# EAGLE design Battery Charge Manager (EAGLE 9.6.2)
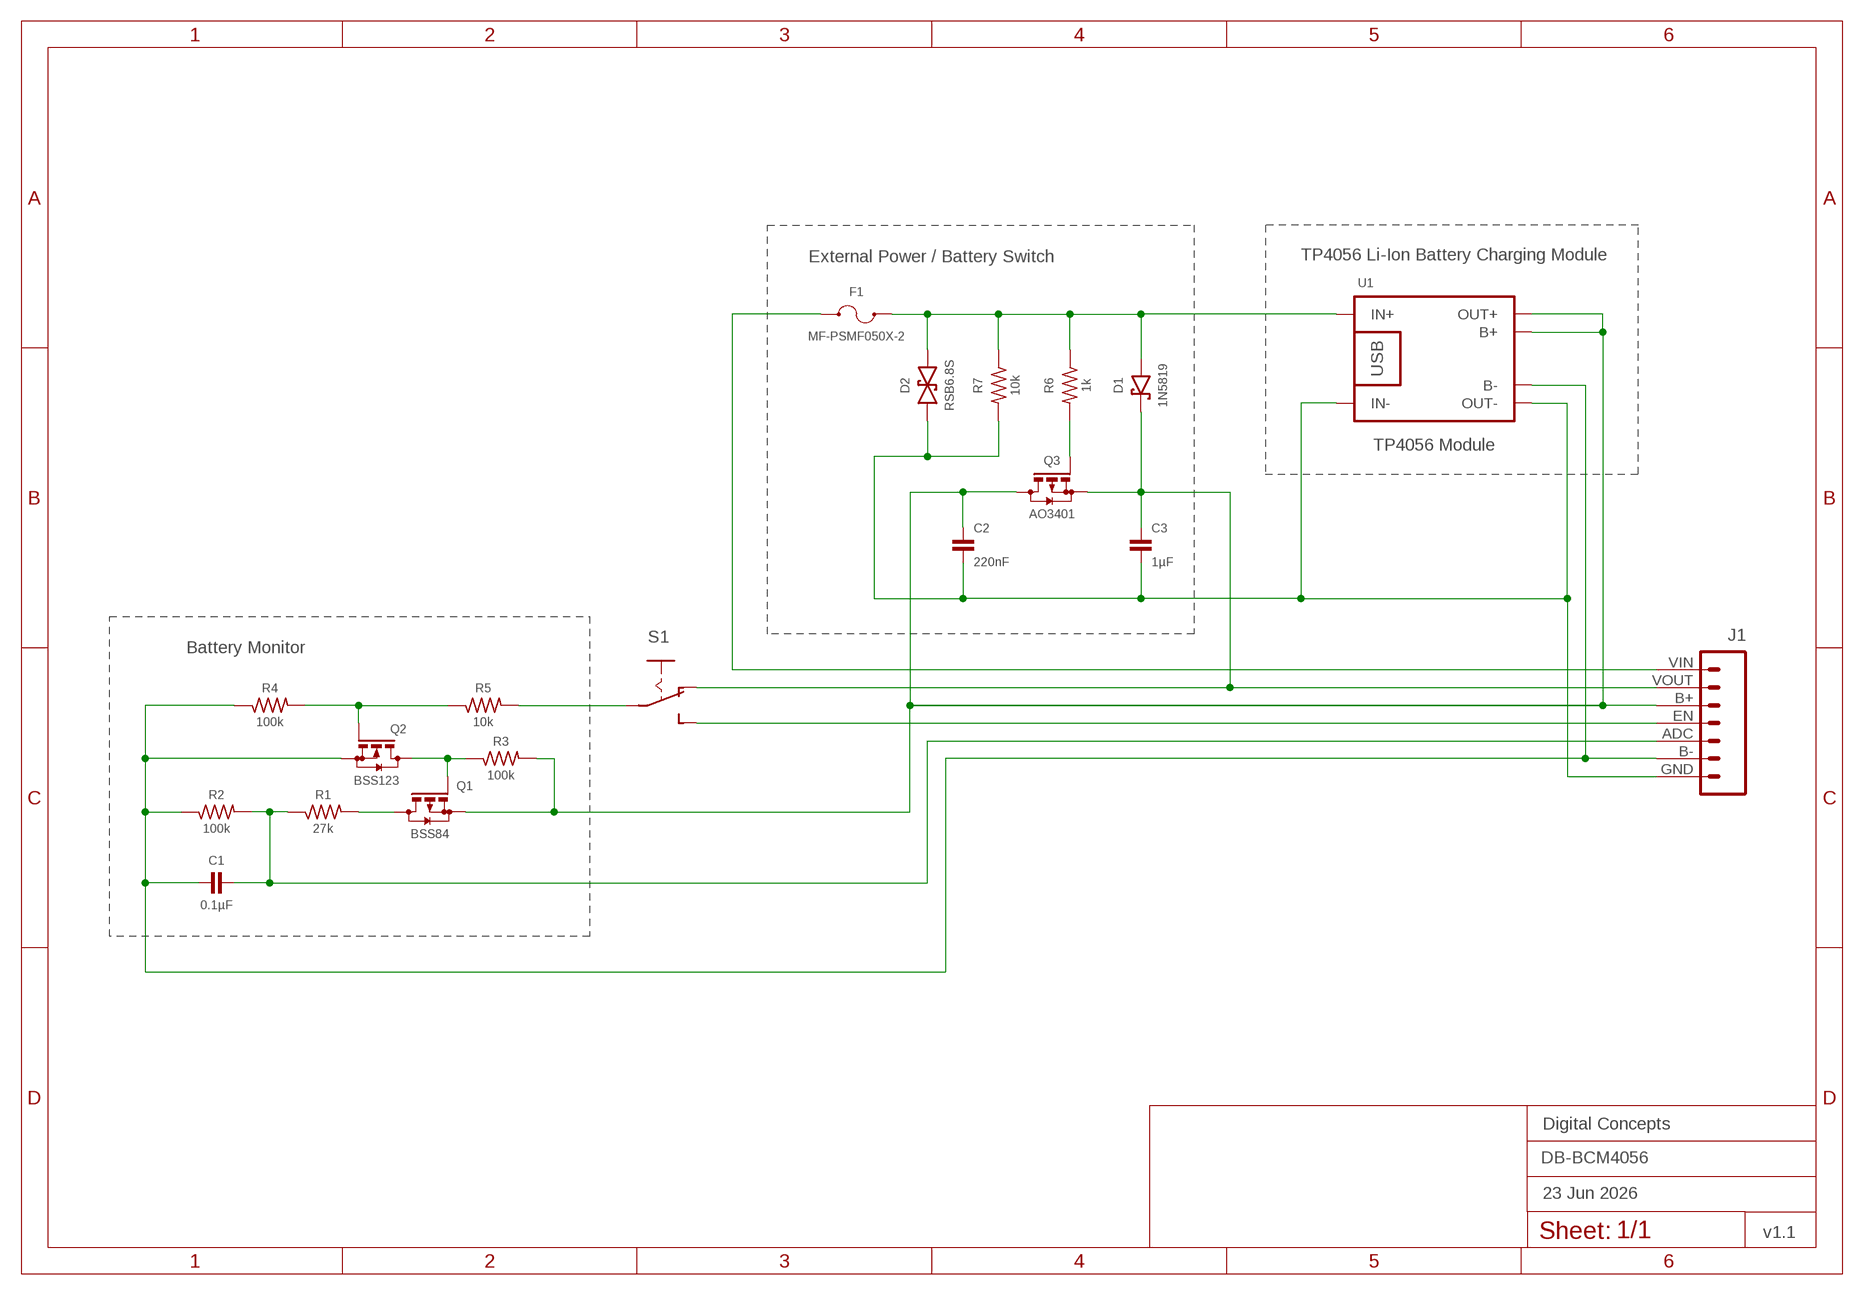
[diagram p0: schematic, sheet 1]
FRAME2 (FRAME-A4L-LOC): DATE: 23 Jun 2026; OWNER: Digital Concepts; TITLE: DB-BCM4056; VERSION: v1.1

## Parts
C1  0.1µF  CAPACITOR-0805  [C0805]
C2  220nF  CAPACITOR-0805  [C0805]
C3  1µF  CAPACITOR-0805  [C0805]
D1  1N5819  DIODE-SCHOTTKY-1N5819  [SOD-123]
D2  RSB6.8S  DIODE-BIDIRECTIONAL-RSB6.8S  [EMD2]
F1  MF-PSMF050X-2  [F0805]
J1  HEADER-1X7-BCS  [CONN_07-BCS]
Q1  BSS84  MOSFET-AO3401  [SOT23-3]
Q2  BSS123  MOSFET-BSS123  [SOT23-3]
Q3  AO3401  MOSFET-AO3401  [SOT23-3]
R1  27k  RESISTORR0805  [R0805]
R2  100k  RESISTORR0805  [R0805]
R3  100k  RESISTORR0805  [R0805]
R4  100k  RESISTORR0805  [R0805]
R5  10k  RESISTORR0805  [R0805]
R6  1k  RESISTORR0805  [R0805]
R7  10k  RESISTORR0805  [R0805]
S1  SWITCH-SLIDE-SPDT-SMT  [SWITCH-SPDT-SMT]
U1  TP4056 Module  TP4056-MODULE-SMALL  [TP4056-MODULE]

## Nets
ADC: C1.1 J1.ADC R1.1 R2.2
B+: C2.1 J1.B+ Q1.2(S) Q3.3(D) R3.2 U1.B+ U1.OUT+
B-: C1.2 J1.B- Q2.2(S) R2.1 R4.1 U1.B-
EN: J1.EN S1.3(S)
GND: C2.2 C3.2 D2.P$2 J1.GND R7.2 U1.IN- U1.OUT-
N$1: Q1.3(D) R1.2
N$2: Q1.1(G) Q2.3(D) R3.1
N$3: Q2.1(G) R4.2 R5.1
N$4: Q3.1(G) R6.2
N$5: D1.A D2.P$1 F1.2 R6.1 R7.1 U1.IN+
N$6: R5.2 S1.2(P)
VIN: F1.1 J1.VIN
VOUT: C3.1 D1.C J1.VOUT Q3.2(S) S1.1(O)

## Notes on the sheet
- External Power / Battery Switch | TP4056 Li-Ion Battery Charging Module
- Battery Monitor

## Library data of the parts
C1-C3 = digitalconcepts:CAPACITOR-0805: 0805 Capacitor
D1 = digitalconcepts:DIODE-SCHOTTKY-1N5819: 1N5819 Schottky Diode SOD-123
D2 = digitalconcepts:DIODE-BIDIRECTIONAL-RSB6.8S: Schottky Bidirectional Diode
F1 = digitalconcepts:MF-PSMF050X-2: PTC Resettable Fuse
J1 = digitalconcepts:HEADER-1X7-BCS: Single Row 7-Pin Header BCS Pin labels
Q1 Q3 = digitalconcepts:MOSFET-AO3401: AO3401 P-Channel MOSFET
Q2 = digitalconcepts:MOSFET-BSS123: N-CHANNEL MOS FET
R1-R7 = digitalconcepts:RESISTOR: Resistor; SPICEPREFIX: R
S1 = digitalconcepts:SWITCH-SLIDE-SPDT-SMT: Mini Sliding Switch SPDT SMT
U1 = digitalconcepts:TP4056-MODULE-SMALL: Lithium Battery 5V Charger with protection circuit TP4056 Li Battery Charger module with PCB (smaller text) footprint More details available here: http://www.instructables.com/id/DIY-Lithium-ion-Battery-Charger/step4/TP4056-based-lithium-ion-battery-charger-module/ Click here to find device on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

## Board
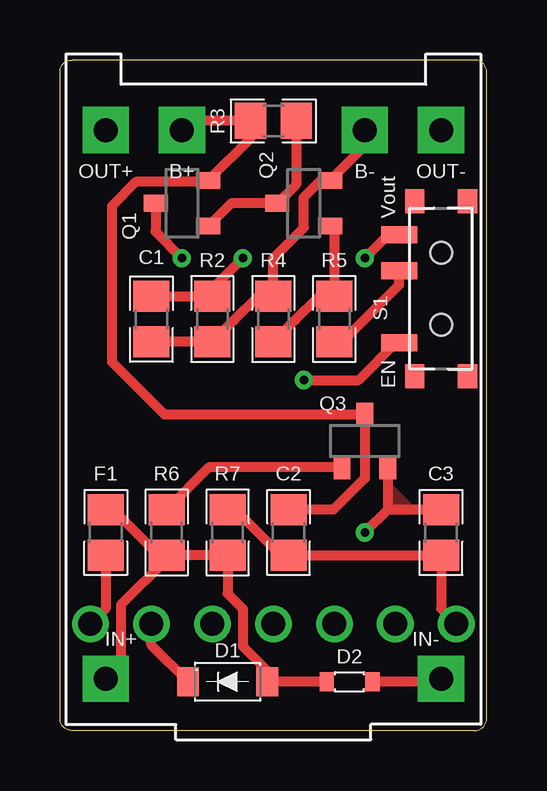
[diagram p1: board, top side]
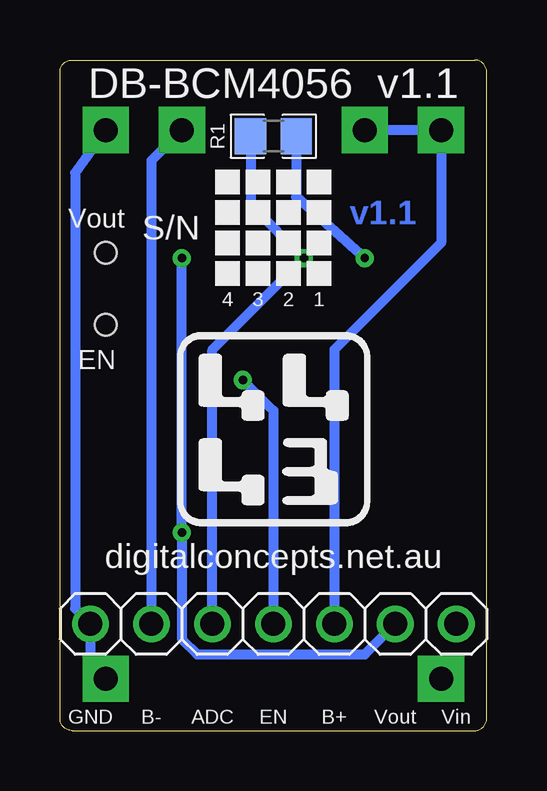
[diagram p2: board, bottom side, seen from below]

Size 17.78 x 27.94 mm. Coordinates in mm from the lower left corner, seen from the top.
Outline: 17.78,27.43 arc90 17.27,27.94 0.51,27.94 arc90 0,27.43 0,0.51 arc90 0.51,0 17.27,0 arc90 17.78,0.51 17.78,27.43
Copper layers (1*16): Top 0.035mm / dielectric 1.5mm / Bottom 0.035mm
Design rules "default *": minimum track width 6mil, minimum drill 0.3mm, track to track 6mil, track to pad 6mil, pad to pad 6mil, via to via 6mil, smd to smd 6mil, copper to edge 6mil, drill to drill 6mil, minimum pad ring 1mil, minimum via ring 8mil, stop-mask expansion 4mil, vias tented up to drill 0mil, thermal gap 10mil

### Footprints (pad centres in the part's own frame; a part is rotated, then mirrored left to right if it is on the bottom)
C0805 = smd 1.3 x 1.5: 1 -0.95,0; 2 0.95,0
SOD-123 = smd 0.91 x 1.22: A -1.65,0; C 1.65,0
EMD2 = smd 0.6 x 0.8: P$1 -0.95,0; P$2 0.95,0
F0805 = smd 1.3 x 1.5: 1 -0.95,0; 2 0.95,0
CONN_07-BCS = drill 1 pad 1.524: ADC 5.08,0; B+ 10.16,0; B- 2.54,0; EN 7.62,0; GND 0,0; VIN 15.24,0; VOUT 12.7,0
SOT23-3 = smd 0.7 x 1: 1 -0.95,-1.1; 2 0.95,-1.1; 3 0,1.1
R0805 = smd 1.3 x 1.5: 1 -0.95,0; 2 0.95,0
SWITCH-SPDT-SMT = smd 0.7 x 1.5: 1 2.25,1.75; 2 0.75,1.75; 3 -2.25,1.75 | smd 1 x 0.8: GND@1 3.65,-1.1; GND@2 3.65,1.1; GND@3 -3.65,1.1; GND@4 -3.65,-1.1 | hole 0.9: -1.5,0; 1.5,0
TP4056-MODULE = drill 1 pad 1.93 square: B+ -10.795,-3.81; B- -10.795,3.81; IN+ 12.065,-6.985; IN- 12.065,6.985; OUT+ -10.795,-6.985; OUT- -10.795,6.985

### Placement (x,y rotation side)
C1  3.81,17.14 270 top
C2  9.53,8.25 270 top
C3  15.88,8.25 270 top
D1  6.99,2.03 180 top
D2  12.06,2.03 0 top
F1  1.91,8.25 90 top
J1  16.51,4.45 0 bottom
Q1  5.08,21.97 90 top
Q2  10.16,21.97 90 top
Q3  12.7,12.06 0 top
R1  8.89,24.77 0 bottom
R2  6.35,17.14 90 top
R3  8.89,25.4 180 top
R4  8.89,17.14 270 top
R5  11.43,17.14 270 top
R6  4.45,8.25 90 top
R7  6.99,8.25 90 top
S1  15.88,18.42 90 top
U1  8.89,14.22 270 top

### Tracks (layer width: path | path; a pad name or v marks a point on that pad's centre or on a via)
ADC  (via drill 0.35)
  Top 0.406: v7.62,19.69 6.35,18.42 R2.2 C1.1
  Bottom 0.406: J1.ADC 11.43,15.87 v7.62,19.69 9.84,21.91 R1.1
B+
  Top 0.406: C2.1 11.39,9.21 12.7,10.51 Q3.3 4.36,13.17 2.16,15.37 2.16,21.85 3.17,22.86 6.12,22.86 Q1.2 7.96,24.7 7.96,25.38 R3.2 5.46,25.4 U1.B+
  Bottom 0.406: U1.B+ U1.OUT+ 1.91,20.32 6.35,15.87 J1.B+
B-
  Top 0.406: C1.2 R2.1 7.24,17.09 7.25,17.09 8.25,18.1 R4.1 8.89,19.69 10.16,20.96 10.16,22.23 10.86,22.92 Q2.2 12.7,24.36 U1.B-
  Bottom 0.406: U1.B- 13.97,23.75 J1.B-
EN  (via drill 0.35)
  Top 0.406: S1.3 14,16.17 12.44,14.6 v10.16,14.6
  Bottom 0.406: v10.16,14.6 8.89,13.33 J1.EN
GND
  Top 0.406: R7.2 7.29,9.21 9.19,7.3 C2.2 C3.2 15.88,5.08 J1.GND | U1.IN- 15.75,2.03 D2.P$2
  Bottom 0.406: U1.OUT- 17.15,23.24 17.15,5.08 J1.GND 16.51,2.79 U1.IN-
N$1  (via drill 0.35)
  Top 0.406: Q1.3 3.98,20.79 v5.08,19.69
  Bottom 0.406: R1.2 7.94,22.24 v5.08,19.69
N$2
  Top 0.406: Q1.1 7.13,21.97 Q2.3 9.84,22.75 R3.1
N$3
  Top 0.406: Q2.1 11.43,20.85 R5.1 10.79,18.1 9.79,17.09 9.78,17.09 R4.2
N$4
  Top 0.406: Q3.1 6.21,10.96 R6.2
N$5
  Top 0.406: R6.1 R7.1 6.99,5.71 7.62,5.07 7.62,3.51 8.63,2.49 D1.A D2.P$1 | F1.2 2.21,9.21 4.11,7.3 R6.1 | R6.1 4.45,7.14 2.54,5.23 2.54,2.79 U1.IN+
N$6
  Top 0.406: R5.2 11.74,16.51 12.06,16.51 14.13,18.57 S1.2
VIN
  Top 0.406: F1.1 1.91,5.08 J1.VIN
VOUT  (via drill 0.35)
  Top 0.406: D1.C 3.81,3.56 J1.VOUT | Q3.2 13.65,9.21 | 13.65,9.21 v12.7,8.25 | C3.1 13.65,9.21 | v12.7,19.69 13.68,20.67 S1.1
  Bottom 0.406: J1.VOUT 5.08,3.18 12.06,3.18 12.7,3.81 v12.7,8.25 v12.7,19.69
  pour Top (no thermals): 13.65,9.21 14.6,9.21 13.65,10.16

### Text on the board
Bottom: v1.1
bPlace: DB-BCM4056 v1.1 | S/N | 1 | 2 | 3 | 4 | digitalconcepts.net.au | Vin | Vout | B+ | EN | ADC | B- | GND
tNames: Vout | EN
bNames: Vout | EN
